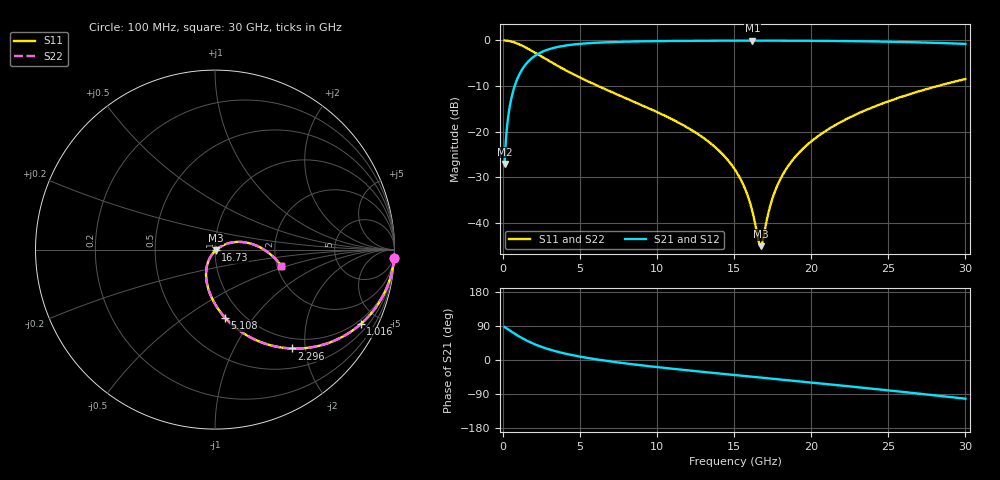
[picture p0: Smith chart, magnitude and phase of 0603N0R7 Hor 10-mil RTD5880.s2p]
# GHz S MA R 50
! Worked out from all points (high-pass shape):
!   3201 points, 100 MHz to 30 GHz, reference 50 ohm
!   highest |S21| = -0.05 dB at 16.18 GHz (marker M1); lowest = -27.1 dB at 100 MHz (marker M2)
!   |S21| within 3 dB of the highest: 2.221 GHz to end of sweep
!   lowest |S11| = -45.1 dB at 16.71 GHz (marker M3), VSWR 1.01, Z = 50.4 - j0.409 ohm
!   |S11| at or under -10 dB: 6.175 GHz to 28.19 GHz (22.01 GHz wide, 128 % of centre)
!   |S22| runs from -45.1 to 0.0 dB; largest |S21 - S12| = 0
!   S11 on the Smith chart (normalised r, x): 100 MHz: 1, -41; 1.016 GHz: 0.81, -3.99; 2.296 GHz: 0.81, -1.74; 5.108 GHz: 0.82, -0.73; 16.73 GHz: 1.01, -0.01; 30 GHz: 2.10, -0.43
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0.1  0.9989 -2.8  0.04429 87.1  0.04429 87.1  0.9989 -2.8
0.4644063  0.9793 -12.9  0.2014 77.0  0.2014 77.0  0.9793 -12.9
1.015688  0.9114 -27.1  0.4106 62.8  0.4106 62.8  0.9114 -27.1
1.595  0.815 -39.9  0.5783 50.0  0.5783 50.0  0.815 -39.9
2.295781  0.6968 -52.2  0.7158 37.6  0.7158 37.6  0.6968 -52.2
3.529156  0.5281 -67.9  0.8472 21.8  0.8472 21.8  0.5281 -67.9
5.089563  0.3853 -81.4  0.9202 8.2  0.9202 8.2  0.3853 -81.4
5.10825  0.3839 -81.5  0.9208 8.1  0.9208 8.1  0.3839 -81.5
10.06978  0.1622 -107.7  0.9827 -19.0  0.9827 -19.0  0.1622 -107.7
13.16256  0.08189 -118.9  0.9918 -32.2  0.9918 -32.2  0.08189 -118.9
15.05  0.03836 -122.1  0.9939 -39.8  0.9939 -39.8  0.03836 -122.1
15.70406  0.0237 -119.4  0.9942 -42.4  0.9942 -42.4  0.0237 -119.4
16.18059  0.01338 -110.3  0.9943 -44.3  0.9943 -44.3  0.01338 -110.3
16.56369  0.006532 -77.7  0.9942 -45.8  0.9942 -45.8  0.006532 -77.7
16.71319  0.005584 -46.6  0.9942 -46.4  0.9942 -46.4  0.005584 -46.6
16.73187  0.005604 -42.3  0.9942 -46.5  0.9942 -46.5  0.005604 -42.3
17.40462  0.01695 21.0  0.9939 -49.1  0.9939 -49.1  0.01695 21.0
17.96525  0.02963 27.1  0.9934 -51.4  0.9934 -51.4  0.02963 27.1
18.84356  0.05028 28.1  0.9923 -54.9  0.9923 -54.9  0.05028 28.1
20.03956  0.07945 25.6  0.9901 -59.7  0.9901 -59.7  0.07945 25.6
25.01978  0.2158 7.6  0.9681 -80.2  0.9681 -80.2  0.2158 7.6
30  0.3777 -13.6  0.9161 -102.1  0.9161 -102.1  0.3777 -13.6
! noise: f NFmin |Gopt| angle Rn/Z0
0.1  0.002891  0.9915  0.3321  0.07816
3.417  0.004114  0.814  10.51  0.004582
6.743  0.00681  0.7825  19.63  0.006243
10.06  0.009288  0.766  28.69  0.007584
13.39  0.0117  0.7565  37.65  0.008722
16.7  0.0141  0.7517  46.38  0.009717
20.03  0.01659  0.7505  54.91  0.01061
23.35  0.0192  0.752  63.19  0.01142
26.67  0.02199  0.7559  71.24  0.01215
30  0.02504  0.7617  79.06  0.01283
